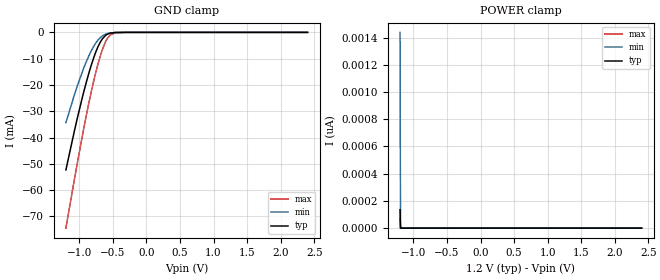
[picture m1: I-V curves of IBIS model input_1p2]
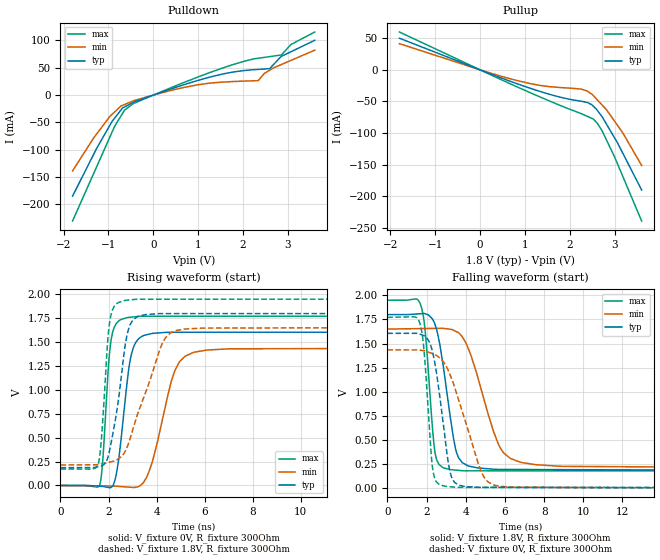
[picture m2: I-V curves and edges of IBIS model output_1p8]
| Texas Instruments Incorporated
| CDCBT1001 1.2V to 1.8V LVCMOS Clock Level Shifter
[IBIS Ver]   4.1
[File name]   cdcbt1001.ibs
[File Rev]   1.0
[Date]   03/16/2022
[Source]
| Texas Instruments Incorporated.
| Analog-eLab Design Center, HPA
| 12500 TI Blvd
| Dallas, TX -75243
[Notes]   Revision History:
| Rev 1.0: 03/16/2022
| - Initial version of the model.
| - Model generated from simulations in SPECTRE.
| - C_comp although listed in numerical order of value are
|   obtained from varying PVT conditions. For PVT conditions for
|   each specific value refer the buffer description under
|   respective [Model]. IBIS model user is responsible for using
|   appropriate C_comp to simulate for Signal Integrity.
[Disclaimer]
| This model is designed as an aid for customers of Texas Instruments.
| TI and its licensors and suppliers make no warranties, either expressed
| or implied, with respect to this  model, including the warranties of
| merchantability or fitness for a particular purpose. The model is
| provided solely on an "as is" basis. The entire risk as to its quality
| and performance is with the customer.
| This model is subject to change without notice. Texas Instruments
| Incorporated is not responsible for updating this model.
[Copyright]
(C) Copyright 2022 Texas Instruments Incorporated.All rights reserved.
|  Component CDCBT1001 5-pin SC70 - DCK Package
|  Part # CDCBT1001
[Component]   CDCBT1001
[Manufacturer]   TI
[Package]   |5 SC70 - DCK Package
|   typ   min   max
R_pkg   0.05   0.04   0.06
L_pkg   1.0nH   0.8nH   1.2nH
C_pkg   0.2pF   0.16pF   0.24pF
[Pin]   signal_name   model_name   R_pin   L_pin   C_pin
1   B   output   NA   NA   NA
2   VCCB   power   NA   NA   NA
3   GND   gnd   NA   NA   NA
4   A   input   NA   NA   NA
5   VCCA   power   NA   NA   NA
|   Model Selectors
[Model Selector]   output
output_1p8   1.8V   Digital Output
[Model Selector]   input
input_1p2   1.2V   Digital Input
| Models and submodels in the file (2): input_1p2 (Input), output_1p8 (Output)
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|   input_1p2 Model
[Model]   input_1p2
Model_type   Input
Vinl = 0.24
Vinh = 0.96
|   typ   min   max
C_comp   1.74pF   1.68pF   1.96pF
[Voltage Range]   1.2   1.08   1.32
[Temperature Range]   27   130   -40
[Power Clamp Reference]   1.2   1.08   1.32
[GND Clamp Reference]   0   0   0
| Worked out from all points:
|   GND clamp passes 1 mA (typ) near -0.60 V on its own axis
[GND Clamp]
|   Voltage   I(typ)   I(min)   I(max)
-1.2V     -52.3mA    -34.31mA   -74.45mA
-1.027V   -32.34mA   -20.17mA   -49.33mA
-926.4mV  -21.88mA   -13.07mA   -35.56mA
-822mV    -12.46mA   -7.005mA   -22.55mA
-750mV    -7.167mA   -3.873mA   -14.74mA
-678mV    -3.299mA   -1.779mA   -8.186mA
-609.6mV  -1.173mA   -698.1uA   -3.591mA
-580.8mV  -685.7uA   -444.5uA   -2.263mA
-537.6mV  -276uA     -212uA     -969.7uA
-465.6mV  -48.27uA   -51.99uA   -160.8uA
-300mV    -352.3nA   -1.074uA   -507.1nA
2.4V      0A         0A         0A
[POWER Clamp]
|   Voltage   I(typ)   I(min)   I(max)
-1.2V     134.9pA    1.438nA    71.79pA
-1.193V   0A         0A         0A
-1.189V   0A         0A         0A
2.4V      0A         0A         0A
|   output_1p8 Model
[Model]   output_1p8
Model_type   Output
Polarity   Non-Inverting
Vmeas = 0.9
Vref = 0
Cref = 2pF
Rref = 100000
|   typ   min   max
C_comp   0.886pF   0.779pF   1.27pF
|  Where Nom  PVT is Nominal Process,   1.8V,  27C
|   Fast PVT is Strong Process,   1.95V, -40C
|   Slow PVT is Weak Process,   1.65V, 130C
[Voltage Range]   1.8   1.65   1.95
|Junction Temperature
[Temperature Range]   27   130   -40
[Pullup Reference]   1.8   1.65   1.95
[Pulldown Reference]   0   -0   -0
[Power Clamp Reference]   1.8   1.65   1.95
[GND Clamp Reference]   0   0   0
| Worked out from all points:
|   slope of the pulldown table from 0 to 0.27 V, typ, clamps not added: 34.8 ohm
|   slope of the pullup table from 0 to 0.27 V, typ, clamps not added: 36.5 ohm
|   falling waveform, V_fixture 1.8V, R_fixture 300Ohm: 20-80 % time 694ps typ, 1.29ns min, 398ps max; typ from 1.8 V to 0.186 V
|   rising waveform, V_fixture 0V, R_fixture 300Ohm: 20-80 % time 437ps typ, 824ps min, 270ps max; typ from 0 V to 1.6 V
|   rising waveform, V_fixture 1.8V, R_fixture 300Ohm: 20-80 % time 544ps typ, 1.15ns min, 279ps max; typ from 0.186 V to 1.8 V
|   falling waveform, V_fixture 0V, R_fixture 300Ohm: 20-80 % time 633ps typ, 1.33ns min, 359ps max; typ from 1.6 V to 0 V
[Pulldown]
|   Voltage   I(typ)   I(min)   I(max)
-1.8V     -184.8mA   -138.7mA   -230.3mA
-1.33V    -108.4mA   -78.37mA   -143.5mA
-918.3mV  -47.94mA   -35.15mA   -67.43mA
-641.6mV  -21.72mA   -17.23mA   -27.53mA
-449.9mV  -13.2mA    -10.59mA   -15.66mA
977mV     26.4mA     18.62mA    32.5mA
1.633V    40.01mA    24.19mA    51.9mA
2.342V    47.03mA    26.61mA    67.47mA
2.594V    48.34mA    45.46mA    70.41mA
2.856V    70.9mA     55.94mA    73.46mA
3.071V    79.39mA    63.54mA    92.68mA
3.6V      100.3mA    82.22mA    115.4mA
[Pullup]
|   Voltage   I(typ)   I(min)   I(max)
-1.8V     50.14mA    41.51mA    59.93mA
778.3mV   -20.75mA   -16.09mA   -25.42mA
1.324V    -33.87mA   -24.45mA   -42.52mA
2.25V     -49.58mA   -30.33mA   -69.16mA
2.393V    -51.63mA   -33.95mA   -73.71mA
2.527V    -57.77mA   -41.03mA   -77.98mA
2.615V    -64.34mA   -47.71mA   -84.84mA
2.717V    -73.97mA   -55.48mA   -96.35mA
2.814V    -85.64mA   -62.84mA   -110.7mA
2.994V    -107.3mA   -80.93mA   -137.3mA
3.177V    -131.5mA   -99.4mA    -168.1mA
3.6V      -190.1mA   -151.2mA   -239.2mA
[Ramp]
R_load = 300
|   typ   min   max
dV/dt_r   0.963238/4.35788e-10   0.860231/8.17571e-10   1.06317/2.69098e-10
dV/dt_f   0.96847/6.93404e-10   0.861348/1.28076e-09   1.06704/3.97377e-10
[Falling Waveform]
V_fixture = 1.8V
V_fixture_min = 1.65V
V_fixture_max = 1.95V
R_fixture = 300Ohm
C_fixture = 0F
|   Time   V(typ)   V(min)   V(max)
0s        1.8V       1.65V      1.95V
1.67ns    1.809V     1.655V     1.918V
1.925ns   1.809V     1.656V     1.642V
2.44ns    1.693V     1.657V     360mV
3.212ns   735.8mV    1.648V     189.7mV
3.494ns   394.5mV    1.626V     184.4mV
3.828ns   261.4mV    1.567V     178.2mV
5.794ns   191.6mV    404.4mV    177mV
7.549ns   190.3mV    241.2mV    177mV
50ns      185.9mV    214.4mV    171.6mV
[Rising Waveform]
V_fixture = 0V
V_fixture_min = 0V
V_fixture_max = 0V
R_fixture = 300Ohm
C_fixture = 0F
|   Time   V(typ)   V(min)   V(max)
0s        -18.2nV    -108.7nV   -63.42nV
1.619ns   -7.246mV   -3.991mV   -5.117mV
2.122ns   -16.32mV   -5.23mV    1.542V
2.392ns   220mV      -8.819mV   1.712V
2.802ns   1.139V     -16.24mV   1.756V
3.069ns   1.462V     -20.95mV   1.762V
3.677ns   1.581V     140.2mV    1.768V
4.922ns   1.601V     1.281V     1.768V
6.097ns   1.601V     1.415V     1.768V
50ns      1.605V     1.434V     1.772V
[Rising Waveform]
V_fixture = 1.8V
V_fixture_min = 1.65V
V_fixture_max = 1.95V
R_fixture = 300Ohm
C_fixture = 0F
|   Time   V(typ)   V(min)   V(max)
0s        185.9mV    214.4mV    171.6mV
1.559ns   196.2mV    217.2mV    213.4mV
1.699ns   203.7mV    225mV      471.7mV
1.962ns   283.7mV    239.7mV    1.497V
2.062ns   388.6mV    245.3mV    1.73V
2.694ns   1.467V     357.9mV    1.935V
3.004ns   1.727V     578.9mV    1.942V
4.215ns   1.796V     1.472V     1.946V
5.189ns   1.796V     1.635V     1.946V
50ns      1.8V       1.65V      1.95V
[Falling Waveform]
|Gnd
V_fixture = 0V
V_fixture_min = 0V
V_fixture_max = 0V
R_fixture = 300Ohm
C_fixture = 0F
|   Time   V(typ)   V(min)   V(max)
0s        1.605V     1.434V     1.772V
1.636ns   1.6V       1.431V     1.725V
1.871ns   1.581V     1.426V     1.433V
2.329ns   1.395V     1.393V     179mV
2.968ns   483.7mV    1.275V     15.83mV
3.187ns   178.8mV    1.181V     11.91mV
3.421ns   58.89mV    1.054V     7.73mV
4.896ns   5.002mV    125.7mV    4.977mV
5.757ns   4.551mV    15.56mV    4.955mV
50ns      5.57nV     102.5nV    46.29nV
